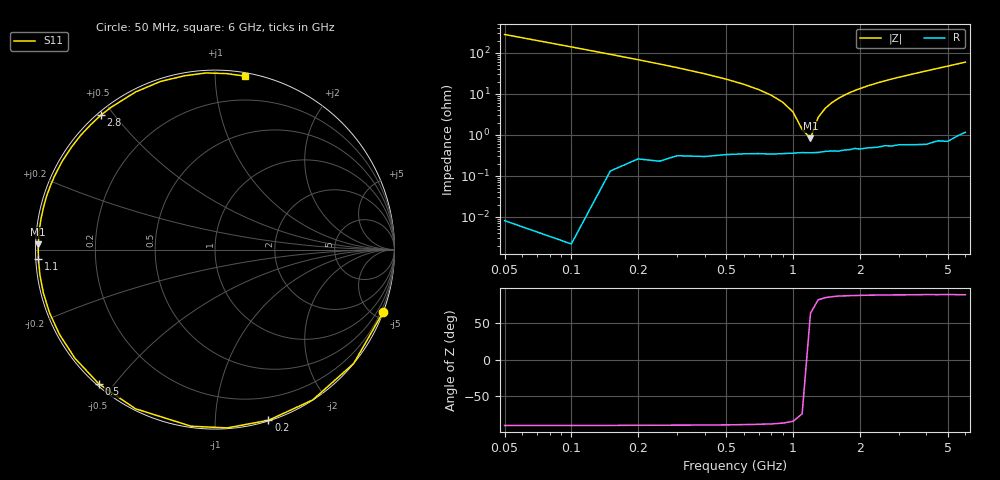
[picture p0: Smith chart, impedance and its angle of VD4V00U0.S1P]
! Infineon Technologies  Discrete & RF Semiconductors
! BBY 55-03
! Si Tuning Diode in SOD323
! VR = 4 V
! S-Parameters:  June  1999
# GHz  S  MA  R  50
!  f  S11
! GHz  MAG  ANG
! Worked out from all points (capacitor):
!   34 points, 50 MHz to 6 GHz, reference 50 ohm
!   read as one part to ground: C = 11.3 pF near 50 MHz
!   lowest |Z| = 828 mohm at 1.2 GHz (marker M1)
!   series resonance near 1.164 GHz, so ESL is about 1.7 nH
!   S11 on the Smith chart (normalised r, x): 50 MHz: 0.00, -5.61; 200 MHz: 0.01, -1.36; 500 MHz: 0.01, -0.46; 1.1 GHz: 0.01, -0.03; 2.8 GHz: 0.01, +0.46; 6 GHz: 0.02, +1.19
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0.05  1 -20.2
0.1  1 -39.4
0.15  0.9988 -57.0
0.2  0.9964 -72.6
0.25  0.9958 -86.1
0.3  0.993 -97.7
0.4  0.9914 -116.6
0.5  0.9891 -130.9
0.6  0.9877 -142.2
0.7  0.9869 -151.4
0.8  0.9869 -159.1
0.9  0.9863 -165.8
1.1  0.9853 -177.0
1.2  0.9854 178.3
1.4  0.9843 169.8
1.6  0.9844 162.5
1.8  0.9835 155.9
2  0.9832 150.0
2.2  0.9825 144.5
2.4  0.9826 139.5
2.8  0.9825 130.4
3  0.9819 126.2
3.5  0.9834 116.7
4  0.9847 108.0
4.5  0.9833 100.0
5  0.9855 92.9
5.5  0.9828 86.1
6  0.9809 80.2
